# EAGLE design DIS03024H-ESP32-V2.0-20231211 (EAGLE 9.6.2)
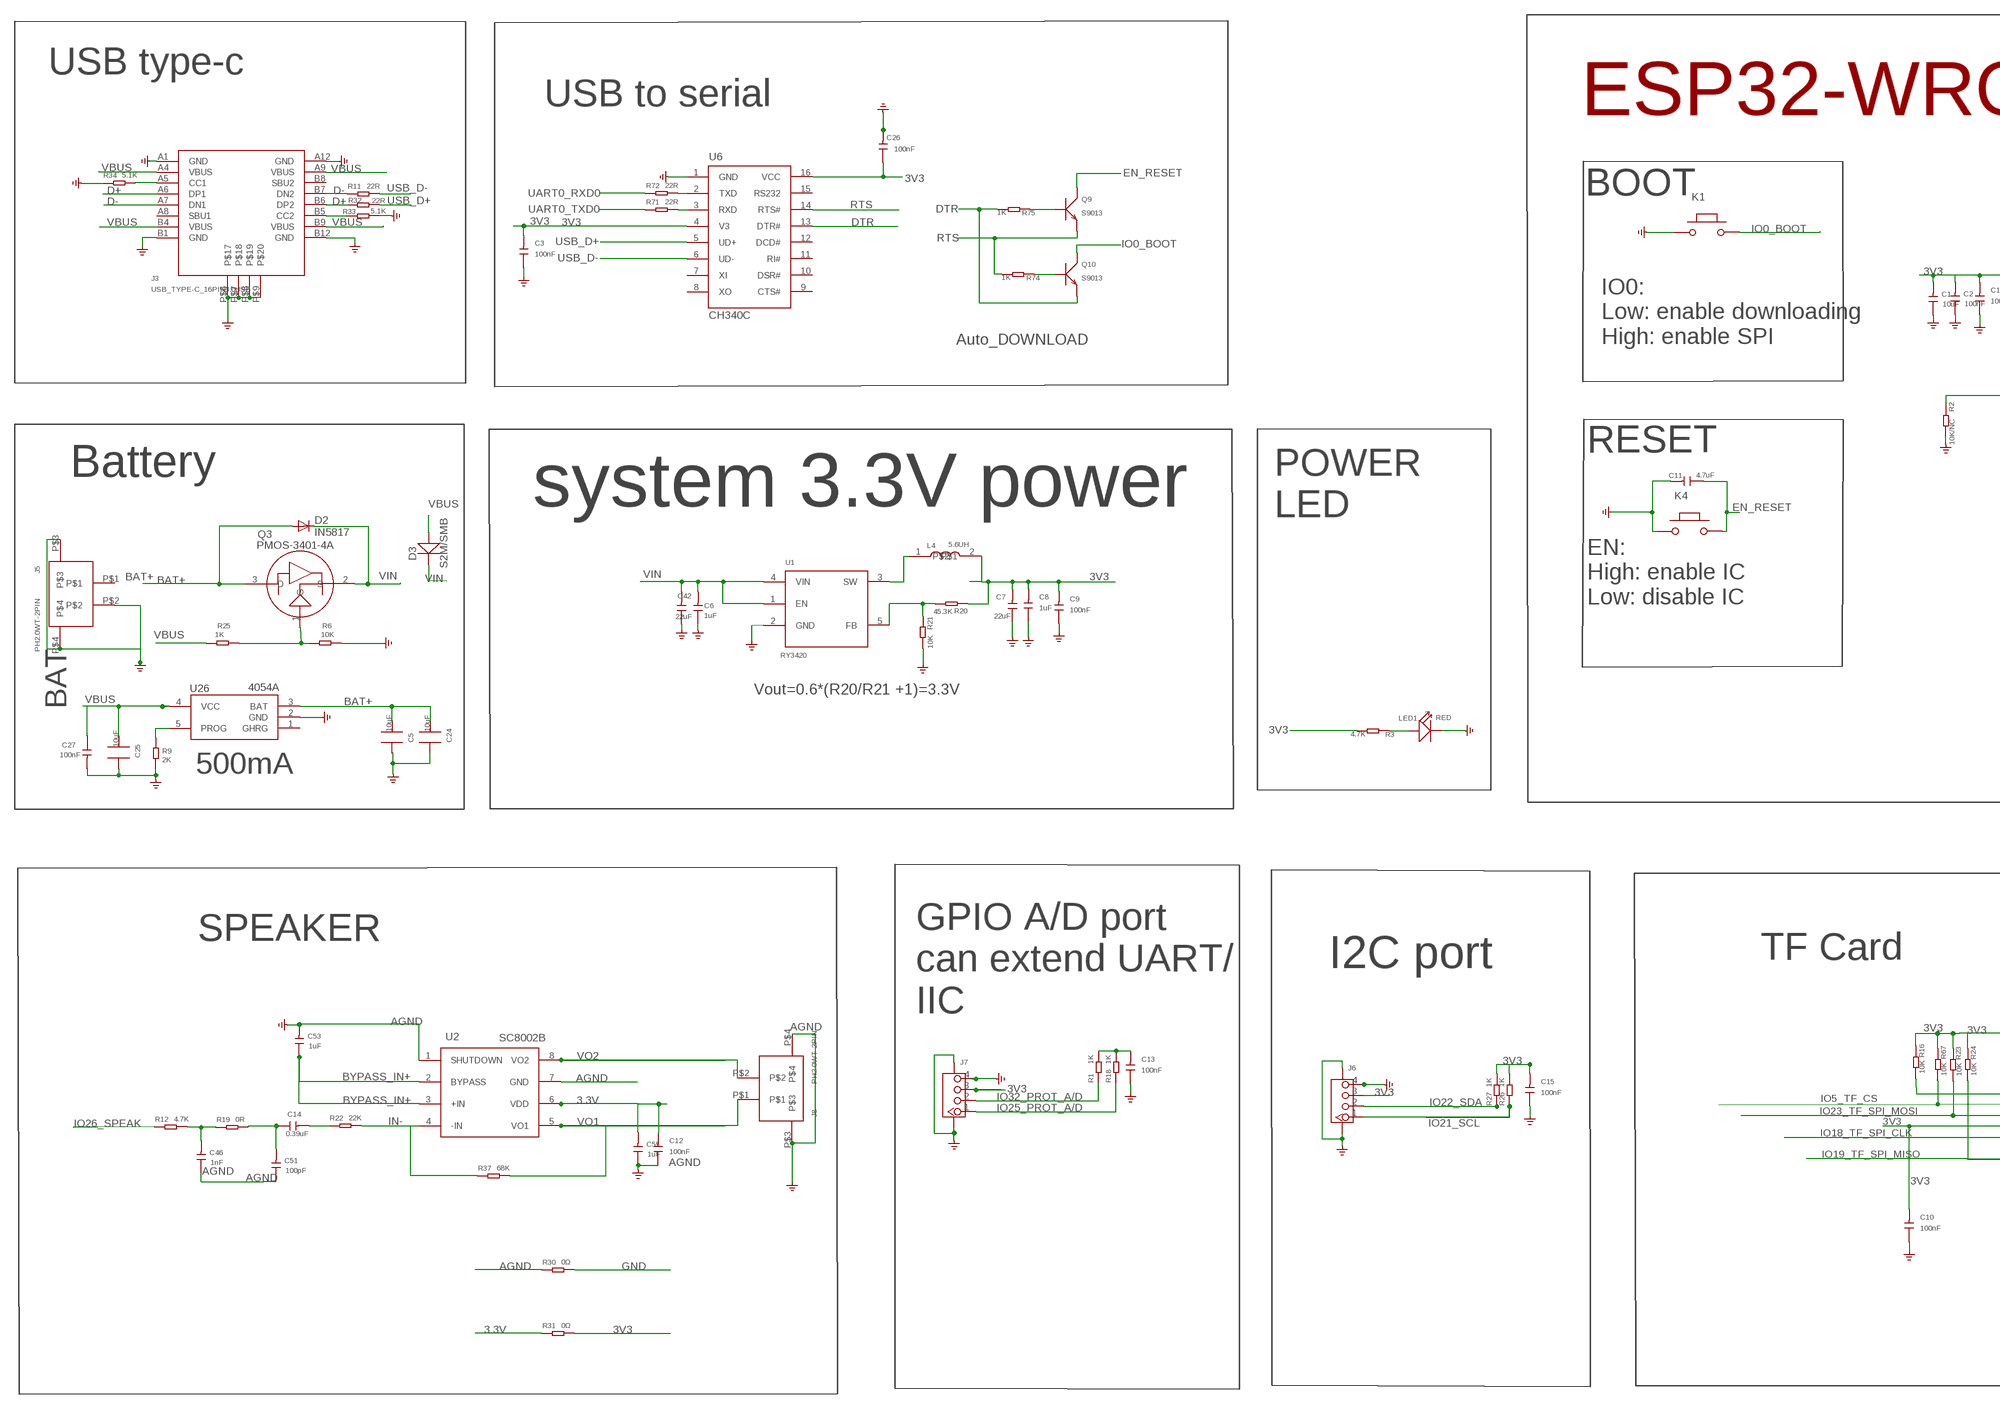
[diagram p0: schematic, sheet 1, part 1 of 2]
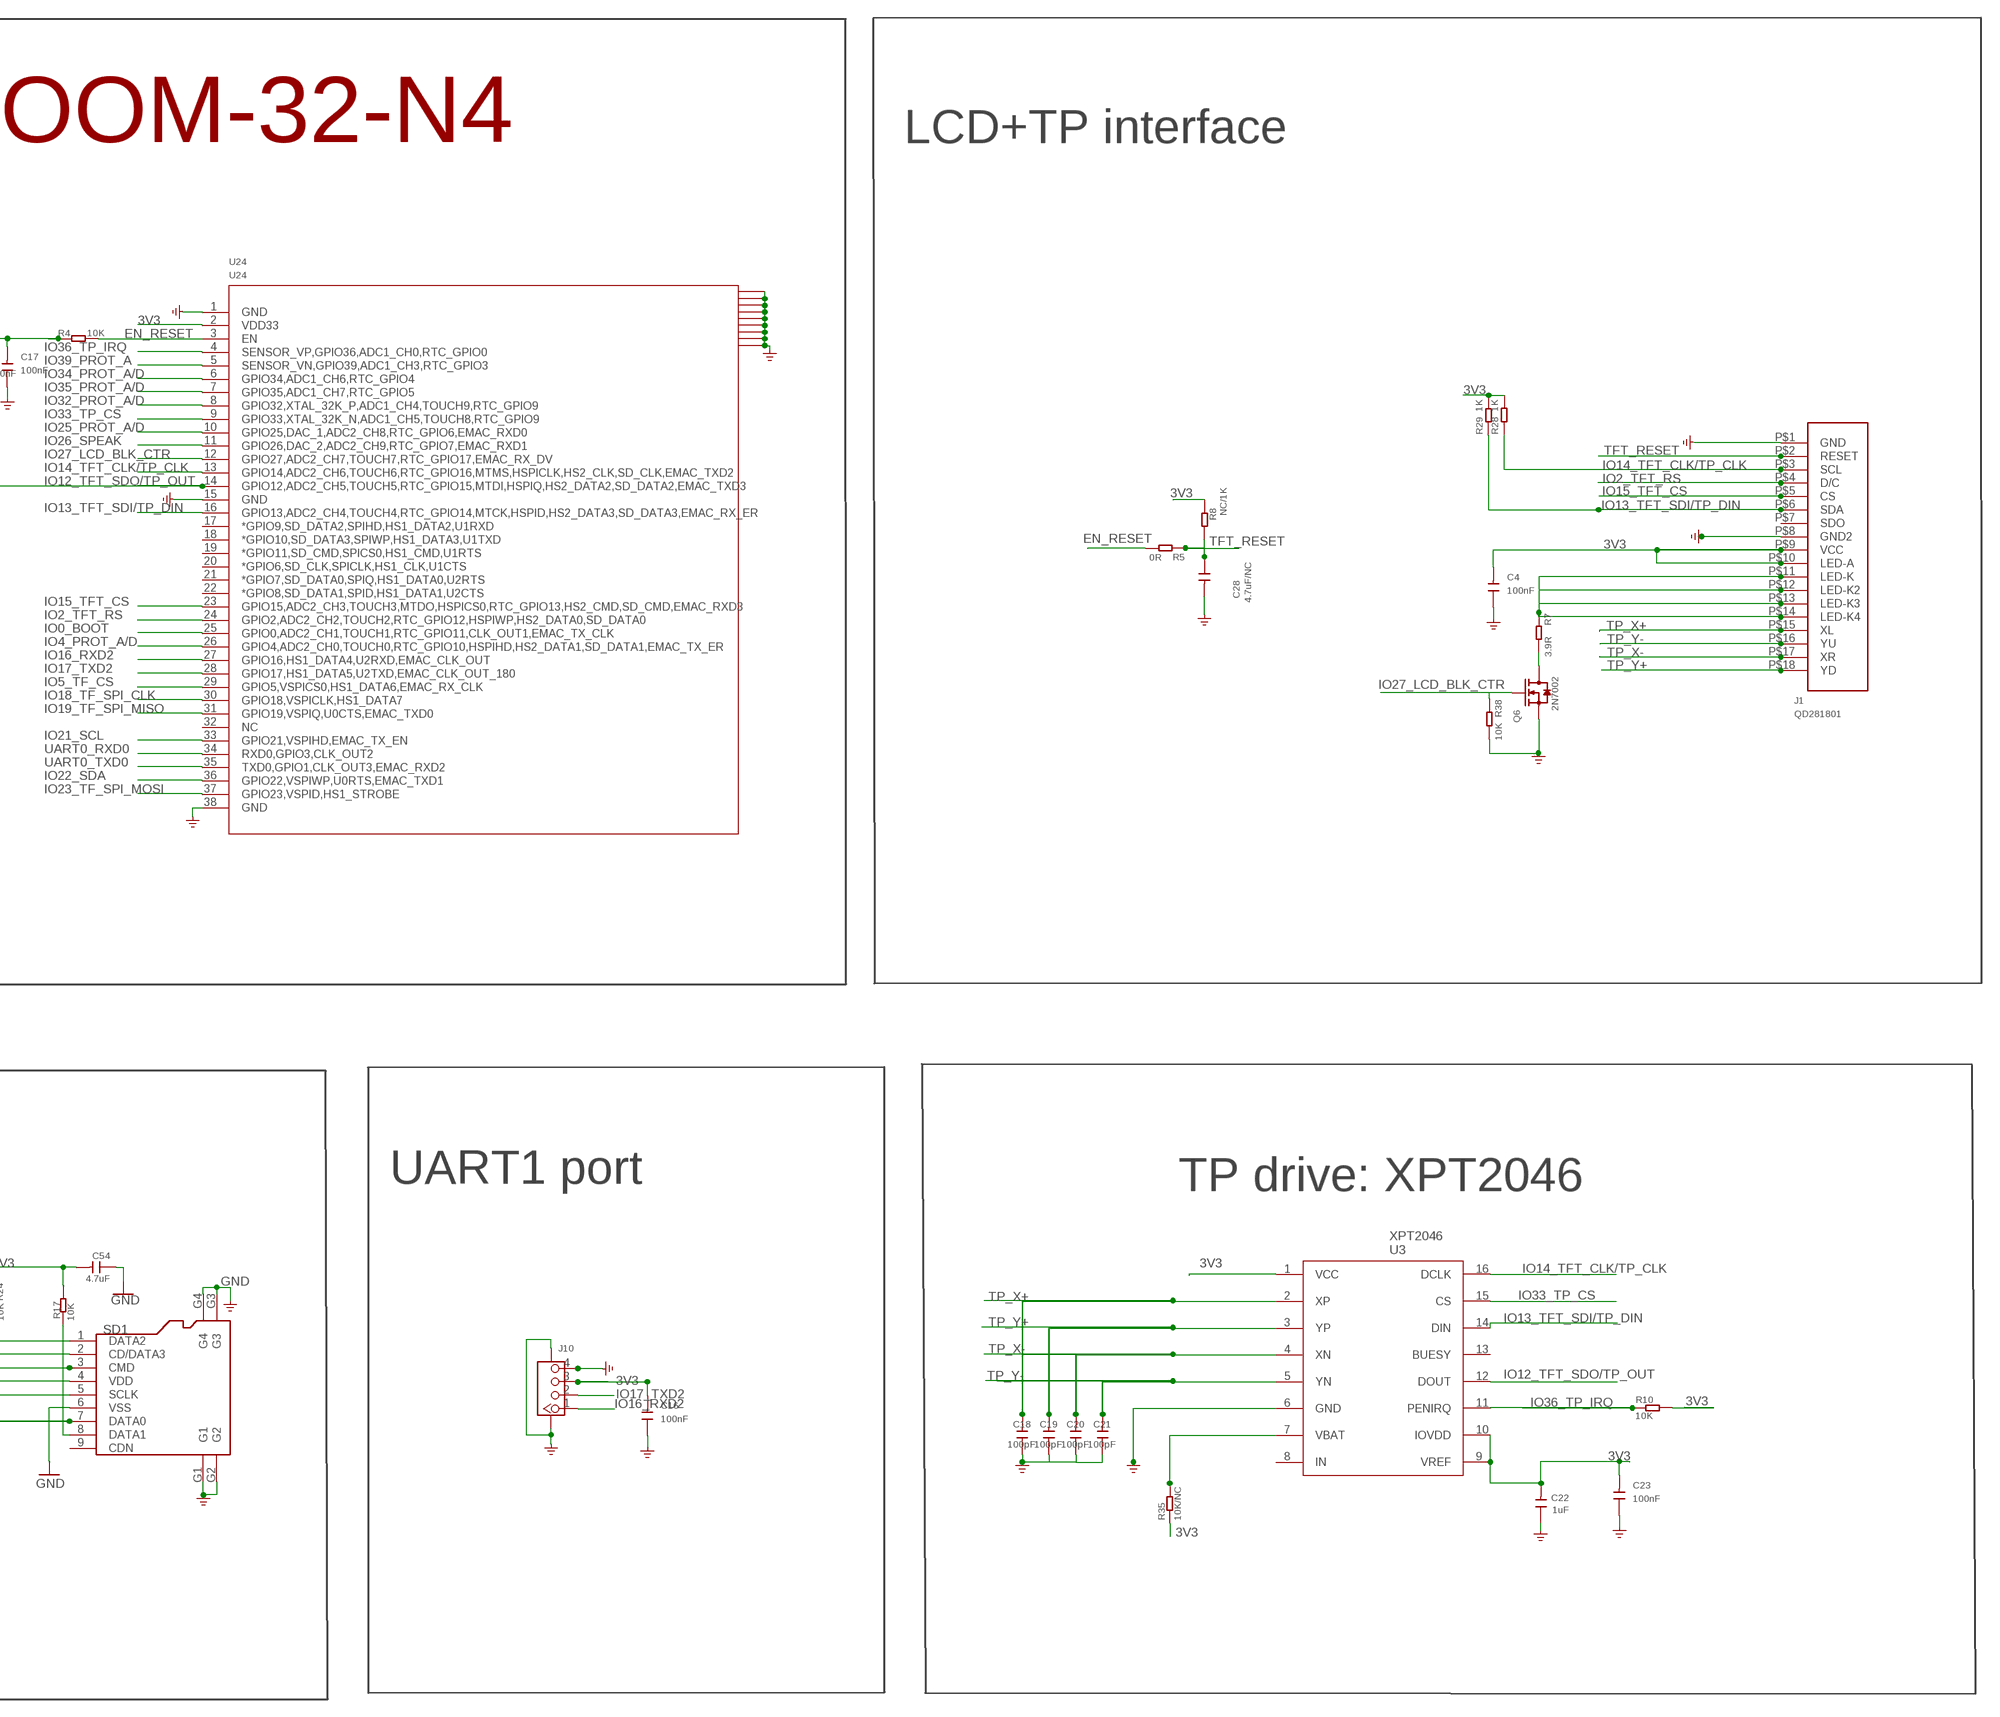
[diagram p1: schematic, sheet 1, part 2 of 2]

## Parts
C1  10uF  DISCRETE_C-0603  [DISCRETE_C0603]
C2  100nF  DISCRETE_C-0603  [DISCRETE_C0603]
C3  100nF  C0603  [0603]
C4  100nF  C0603  [0603]
C5  10uF  C0805_S  [0805_S]
C6  1uF  C0603  [0603]
C7  22uF  C0805  [0805]
C8  1uF  C0603  [0603]
C9  100nF  C0603  [0603]
C10  100nF  C0603  [0603]
C11  4.7uF  C0603  [0603]
C12  100nF  C0603  [0603]
C13  100nF  C0603  [0603]
C14  0.39uF  DISCRETE_C-0603  [DISCRETE_C0603]
C15  100nF  C0603  [0603]
C16  100nF  C0603  [0603]
C17  100nF  C0603  [0603]
C18  100pF  C0603  [0603]
C19  100pF  C0603  [0603]
C20  100pF  C0603  [0603]
C21  100pF  C0603  [0603]
C22  1uF  DISCRETE_C-0603  [DISCRETE_C0603]
C23  100nF  C0603  [0603]
C24  10uF  C0805_S  [0805_S]
C25  10uF  C0805_S  [0805_S]
C26  100nF  C0603  [0603]
C27  100nF  C-0603  [C0603]
C28  4.7uF/NC  C0603  [0603]
C42  22uF  C0805  [0805]
C46  1nF  DISCRETE_C-0603  [DISCRETE_C0603]
C51  100pF  DISCRETE_C-0603  [DISCRETE_C0603]
C53  1uF  DISCRETE_C-0603  [DISCRETE_C0603]
C54  4.7uF  DISCRETE_C-0603  [DISCRETE_C0603]
C55  1uF  DISCRETE_C-0603  [DISCRETE_C0603]
D2  IN5817  DIODE-DO-214AC  [DO-214AC]
D3  S2M/SMB  214ABDO-214AB  [214AB]
J1  QD281801  [QD241801-18PIN*0.8]
J3  USB_TYPE-C_16PIN3.0USB  [KEVIN_3.0TYPEC-SMD]
J5  PH2.0WT-2PIN  [PH2.0WT-2PIN]
J6  CONNECTOR_TWIG-4P-2.0-SMD-FEMALE-REINFORCE90D  [CONNECTOR_4P-SMD-2.0-90D]
J7  CONNECTOR_TWIG-4P-2.0-SMD-FEMALE-REINFORCE90D  [CONNECTOR_4P-SMD-2.0-90D]
J8  PH2.0WT-2PIN  [PH2.0WT-2PIN]
J10  CONNECTOR_TWIG-4P-2.0-SMD-FEMALE-REINFORCE90D  [CONNECTOR_4P-SMD-2.0-90D]
K1  BUTTON  PB157  [157SW]
K4  BUTTON  PB157  [157SW]
L4  5.6UH  L-0530  [CD54_CD54]
LED1  RED  DISCRETE_LED0603  [DISCRETE_LED-0603]
Q3  PMOS-3401-4A  P-MOS-SOT23  [SOT-23]
Q6  2N7002  MOSFET-N'SOT23'  [SOT23]
Q9  S9013  TRANSISTOR-NPN-SOT23  [SOT23@1]
Q10  S9013  TRANSISTOR-NPN-SOT23  [SOT23@1]
R1  1K  DISCRETE_R-0603  [DISCRETE_R0603]
R2  10K/NC  DISCRETE_R-0603  [DISCRETE_R0603]
R3  4.7K  DISCRETE_R-0603  [DISCRETE_R0603]
R4  10K  R0603  [R0603]
R5  0R  DISCRETE_R-0603  [DISCRETE_R0603]
R6  10K  DISCRETE_R-0603  [DISCRETE_R0603]
R7  3.9R  DISCRETE_R-0603  [DISCRETE_R0603]
R8  NC/1K  DISCRETE_R-0603  [DISCRETE_R0603]
R9  2K  DISCRETE_R-0603  [DISCRETE_R0603]
R10  10K  DISCRETE_R-0603  [DISCRETE_R0603]
R11  22R  DISCRETE_R-0603  [DISCRETE_R0603]
R12  4.7K  DISCRETE_R-0603  [DISCRETE_R0603]
R16  10K  DISCRETE_R-0603  [DISCRETE_R0603]
R17  10K  DISCRETE_R-0603  [DISCRETE_R0603]
R18  1K  DISCRETE_R-0603  [DISCRETE_R0603]
R19  0R  DISCRETE_R-0603  [DISCRETE_R0603]
R20  45.3K  DISCRETE_R-0603  [DISCRETE_R0603]
R21  10K  DISCRETE_R-0603  [DISCRETE_R0603]
R22  22K  DISCRETE_R-0603  [DISCRETE_R0603]
R23  10K  DISCRETE_R-0603  [DISCRETE_R0603]
R24  10K  DISCRETE_R-0603  [DISCRETE_R0603]
R25  1K  DISCRETE_R-0603  [DISCRETE_R0603]
R26  1K  DISCRETE_R-0603  [DISCRETE_R0603]
R27  1K  DISCRETE_R-0603  [DISCRETE_R0603]
R28  1K  DISCRETE_R-0603  [DISCRETE_R0603]
R29  1K  DISCRETE_R-0603  [DISCRETE_R0603]
R30  0Ω  DISCRETE_R-0603  [DISCRETE_R0603]
R31  0Ω  DISCRETE_R-0603  [DISCRETE_R0603]
R32  22R  DISCRETE_R-0603  [DISCRETE_R0603]
R33  5.1K  DISCRETE_R-0603  [DISCRETE_R0603]
R34  5.1K  DISCRETE_R-0603  [DISCRETE_R0603]
R35  10K/NC  DISCRETE_R-0603  [DISCRETE_R0603]
R37  68K  DISCRETE_R-0603  [DISCRETE_R0603]
R38  10K  DISCRETE_R-0603  [DISCRETE_R0603]
R67  10K  DISCRETE_R-0603  [DISCRETE_R0603]
R71  22R  DISCRETE_R-0603  [DISCRETE_R0603]
R72  22R  DISCRETE_R-0603  [DISCRETE_R0603]
R74  1K  DISCRETE_R-0603  [DISCRETE_R0603]
R75  1K  DISCRETE_R-0603  [DISCRETE_R0603]
SD1  HOLDER-MICROSD-9P  [9P-SMD-W/-RING]
U1  RY3420  A_XBJ_HM3420B  [A_XBJ_SOT23-5]
U2  SC8002B  SC8002BSC8002B-SOP8  [AT24C02_SOP8]
U3  XPT2046  [XP2046-SSOP16]
U6  CH340C  CH340G  [SOP-16]
U24  U24  ESP32-WROOM-32-N4  [ESP32-WROOM-32-N4]
U26  4054A  [SOP23-5]

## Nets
3.3V: C12.2 C55.2 R31.1 U2.6(VDD)
3V3: C1.2 C2.2 C3.2 C4.2 C7.2 C8.2 C9.2 C10.2 C13.2 C15.2 C16.2 C17.2 C22.2 C23.2 C26.1 C54.2 J1.P$9(VCC) J1.P$10(LED-A) J6.3 J7.3 J10.3 L4.2 R1.2 R3.2 R4.1 R8.2 R10.2 R16.1 R17.1 R18.2 R20.1 R23.1 R24.1 R26.2 R27.2 R28.2 R29.2 R31.2 R35.1 R67.1 SD1.4(VDD) U3.1(VCC) U3.9(VREF) U3.10(IOVDD) U6.4(V3) U6.16(VCC) U24.2(VDD33)
AGND: C12.1 C46.1 C51.1 C53.2 C55.1 J8.P$3 J8.P$4 R30.1 U2.1(SHUTDOWN) U2.7(GND) ; supply symbol labelled GND
BAT+: C5.2 C24.2 D2.A J5.P$1 Q3.3(D) U26.3(BAT)
BYPASS_IN+: C53.1 U2.2(BYPASS) U2.3(+IN)
D+: J3.A6(DP1) J3.B6(DP2) R32.1
D-: J3.A7(DN1) J3.B7(DN2) R11.1
DTR: Q10.2(E) R75.2 U6.13(DTR#)
EN_RESET: C11.1 K4.2 Q9.3(C) R4.2 R5.2 U24.3(EN)
GND: C1.1 C2.1 C3.1 C4.1 C5.1 C6.1 C7.1 C8.1 C9.1 C10.1 C11.2 C13.1 C15.1 C16.1 C17.1 C18.1 C19.1 C20.1 C21.1 C22.1 C23.1 C24.1 C25.1 C26.2 C27.2 C28.2 C42.1 C54.1 J1.P$1(GND) J1.P$8(GND2) J3.A1(GND) J3.A12(GND) J3.B1(GND) J3.B12(GND) J3.P$6 J3.P$7 J3.P$8 J3.P$9 J5.P$2 J5.P$3 J5.P$4 J6.4 J6.SS1 J6.SS2 J7.4 J7.SS1 J7.SS2 J10.4 J10.SS1 J10.SS2 K1.1 K4.1 LED1.- Q6.2(S) R2.2 R6.1 R9.2 R21.2 R30.2 R33.2 R34.1 R38.2 SD1.6(VSS) SD1.G1 SD1.G2 SD1.G3 SD1.G4 U1.2(GND) U3.6(GND) U6.1(GND) U24.1(GND) U24.15(GND) U24.38(GND) U24.41(GND) U24.42(GND) U24.43(GND) U24.44(GND) U24.45(GND) U24.46(GND) U24.47(GND) U24.48(GND) U24.49(GND) U26.2(GND)
IN-: R22.2 R37.1 U2.4(-IN)
IO0_BOOT: K1.2 Q10.3(C) U24.25(GPIO0,ADC2_CH1,TOUCH1,RTC_GPIO11,CLK_OUT1,EMAC_TX_CLK)
IO2_TFT_RS: J1.P$4(D/C) U24.24(GPIO2,ADC2_CH2,TOUCH2,RTC_GPIO12,HSPIWP,HS2_DATA0,SD_DATA0)
IO4_PROT_A/D: U24.26(GPIO4,ADC2_CH0,TOUCH0,RTC_GPIO10,HSPIHD,HS2_DATA1,SD_DATA1,EMAC_TX_ER)
IO5_TF_CS: R67.2 SD1.2(CD/DATA3) U24.29(GPIO5,VSPICS0,HS1_DATA6,EMAC_RX_CLK)
IO12_TFT_SDO/TP_OUT: R2.1 U3.12(DOUT) U24.14(GPIO12,ADC2_CH5,TOUCH5,RTC_GPIO15,MTDI,HSPIQ,HS2_DATA2,SD_DATA2,EMAC_TXD3)
IO13_TFT_SDI/TP_DIN: J1.P$6(SDA) R29.1 U3.14(DIN) U24.16(GPIO13,ADC2_CH4,TOUCH4,RTC_GPIO14,MTCK,HSPID,HS2_DATA3,SD_DATA3,EMAC_RX_ER)
IO14_TFT_CLK/TP_CLK: J1.P$3(SCL) R28.1 U3.16(DCLK) U24.13(GPIO14,ADC2_CH6,TOUCH6,RTC_GPIO16,MTMS,HSPICLK,HS2_CLK,SD_CLK,EMAC_TXD2)
IO15_TFT_CS: J1.P$5(CS) U24.23(GPIO15,ADC2_CH3,TOUCH3,MTDO,HSPICS0,RTC_GPIO13,HS2_CMD,SD_CMD,EMAC_RXD3)
IO16_RXD2: J10.1 U24.27(GPIO16,HS1_DATA4,U2RXD,EMAC_CLK_OUT)
IO17_TXD2: J10.2 U24.28(GPIO17,HS1_DATA5,U2TXD,EMAC_CLK_OUT_180)
IO18_TF_SPI_CLK: SD1.5(SCLK) U24.30(GPIO18,VSPICLK,HS1_DATA7)
IO19_TF_SPI_MISO: R24.2 SD1.7(DATA0) U24.31(GPIO19,VSPIQ,U0CTS,EMAC_TXD0)
IO21_SCL: J6.1 R26.1 U24.33(GPIO21,VSPIHD,EMAC_TX_EN)
IO22_SDA: J6.2 R27.1 U24.36(GPIO22,VSPIWP,U0RTS,EMAC_TXD1)
IO23_TF_SPI_MOSI: R23.2 SD1.3(CMD) U24.37(GPIO23,VSPID,HS1_STROBE)
IO25_PROT_A/D: J7.1 R18.1 U24.10(GPIO25,DAC_1,ADC2_CH8,RTC_GPIO6,EMAC_RXD0)
IO26_SPEAK: R12.1 U24.11(GPIO26,DAC_2,ADC2_CH9,RTC_GPIO7,EMAC_RXD1)
IO27_LCD_BLK_CTR: Q6.1(G) R38.1 U24.12(GPIO27,ADC2_CH7,TOUCH7,RTC_GPIO17,EMAC_RX_DV)
IO32_PROT_A/D: J7.2 R1.1 U24.8(GPIO32,XTAL_32K_P,ADC1_CH4,TOUCH9,RTC_GPIO9)
IO33_TP_CS: U3.15(CS) U24.9(GPIO33,XTAL_32K_N,ADC1_CH5,TOUCH8,RTC_GPIO9)
IO34_PROT_A/D: U24.6(GPIO34,ADC1_CH6,RTC_GPIO4)
IO35_PROT_A/D: U24.7(GPIO35,ADC1_CH7,RTC_GPIO5)
IO36_TP_IRQ: R10.1 U3.11(PENIRQ) U24.4(SENSOR_VP,GPIO36,ADC1_CH0,RTC_GPIO0)
IO39_PROT_A: U24.5(SENSOR_VN,GPIO39,ADC1_CH3,RTC_GPIO3)
N$1: LED1.+ R3.1
N$2: Q6.3(D) R7.2
N$3: C46.2 R12.2 R19.1
N$4: R35.2 U3.7(VBAT)
N$6: R9.1 U26.5(PROG)
N$12: J1.P$11(LED-K) J1.P$12(LED-K2) J1.P$13(LED-K3) J1.P$14(LED-K4) R7.1
N$13: L4.1 U1.3(SW)
N$14: J3.B5(CC2) R33.1
N$16: J3.A5(CC1) R34.2
N$17: Q3.1(G) R6.2 R25.1
N$20: R20.2 R21.1 U1.5(FB)
N$26: C14.1 C51.2 R19.2
N$29: C14.2 R22.1
N$32: Q9.1(B) R75.1
N$38: Q10.1(B) R74.1
N$40: R72.2 U6.2(TXD)
N$42: R71.2 U6.3(RXD)
N$47: R16.2 SD1.1(DATA2)
N$48: R17.2 SD1.8(DATA1)
RTS: Q9.2(E) R74.2 U6.14(RTS#)
TFT_RESET: C28.1 J1.P$2(RESET) R5.1 R8.1
TP_X+: C18.2 J1.P$15(XL) U3.2(XP)
TP_X-: C20.2 J1.P$17(XR) U3.4(XN)
TP_Y+: C19.2 J1.P$18(YD) U3.3(YP)
TP_Y-: C21.2 J1.P$16(YU) U3.5(YN)
UART0_RXD0: R72.1 U24.34(RXD0,GPIO3,CLK_OUT2)
UART0_TXD0: R71.1 U24.35(TXD0,GPIO1,CLK_OUT3,EMAC_RXD2)
USB_D+: R32.2 U6.5(UD+)
USB_D-: R11.2 U6.6(UD-)
VBUS: C25.2 C27.1 D3.1(+) J3.A4(VBUS) J3.A9(VBUS) J3.B4(VBUS) J3.B9(VBUS) R25.2 U26.4(VCC)
VIN: C6.2 C42.2 D2.C D3.2(-) Q3.2(S) U1.1(EN) U1.4(VIN)
VO1: J8.P$1 R37.2 U2.5(VO1)
VO2: J8.P$2 U2.8(VO2)
Unconnected: J1.P$7(SDO) J3.A8(SBU1) J3.B8(SBU2) SD1.9(CDN) U3.8(IN) U3.13(BUESY) U6.7(XI) U6.8(XO) U6.9(CTS#) U6.10(DSR#) U6.11(RI#) U6.12(DCD#) U6.15(RS232) U24.17(*GPIO9,SD_DATA2,SPIHD,HS1_DATA2,U1RXD) U24.18(*GPIO10,SD_DATA3,SPIWP,HS1_DATA3,U1TXD) U24.19(*GPIO11,SD_CMD,SPICS0,HS1_CMD,U1RTS) U24.20(*GPIO6,SD_CLK,SPICLK,HS1_CLK,U1CTS) U24.21(*GPIO7,SD_DATA0,SPIQ,HS1_DATA0,U2RTS) U24.22(*GPIO8,SD_DATA1,SPID,HS1_DATA1,U2CTS) U24.32(NC) U26.1(GHRG)

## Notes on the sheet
- USB type-c
- USB to serial | ESP32-WROOM-32-N4 | LCD+TP interface
- BOOT
- IO0:
  Low: enable downloading
  High: enable SPI
- Auto_DOWNLOAD
- RESET
- Battery
- system 3.3V power
- POWER
  LED
- EN:
  High: enable IC
  Low: disable IC
- Vout=0.6*(R20/R21 +1)=3.3V
- BAT
- 500mA
- SPEAKER
- I2C port | TF Card | UART1 port
- TP drive: XPT2046
- GPIO A/D port
  can extend UART/
  IIC

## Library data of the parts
C1 C2 C14 C22 C46 C51 C53 C55 = A_xbj:DISCRETE_C*: Ceramic Capacitors
C3 C4 C6 C8-C13 C15-C21 C23 C26 C28 = A_xbj:C0603
C5 C24 C25 = CPT_SMD:C0805
C7 C42 = A_xbj:C0805
C27 = discrete:C*: Ceramic Capacitors
C54 = A9G:DISCRETE_C*: Ceramic Capacitors
D2 = diode:DIODE-: DIODE
D3 = DO-214AB:214AB: 214AB
J1 = cooper:QD281801
J3 = WZ3532R024-ESP32-V0.1-20221226:USB_TYPE-C_16PIN
J5 J8 = cooper:PH2.0WT-2PIN
J6 J7 J10 = A_xbj:CONNECTOR_TWIG-4P-2.0-SMD-FEMALE-REINFORCE
K1 K4 = MySMD:PB157
L4 = WZ2432R028-ESP32-V1.2-20231108:L-0530
LED1 = A_xbj:DISCRETE_LED*
Q3 = DFN8:P-MOS-SOT23
Q6 = discrete:MOSFET-N: IRLL014: http://www.vishay.com/docs/91319/sihll014.pdf
Q9 Q10 = discrete:TRANSISTOR-NPN*: NPN audion
R1-R3 R5 R7 R8 R11 R12 R16-R24 R26-R34 R37 R38 R67 R71 R72 R74 R75 = Crowtail-_LED-V2.0-20190615-01:DISCRETE_R*
R4 = A_xbj:R0603
R6 R9 R10 R25 R35 = A9G:DISCRETE_R*
SD1 = Connector:HOLDER-MICROSD-9P
U1 = CrowBot_-V1.0-20220525:A_XBJ_HM3420B
U2 = cooper:SC8002B
U3 = cooper:XPT2046
U6 = A_xbj:CH340G
U24 = cooper:ESP32-WROOM-32-N4
U26 = DFN8:4054A

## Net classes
0 default: width 0.152 mm, drill 0.305 mm, clearance 0.203 mm

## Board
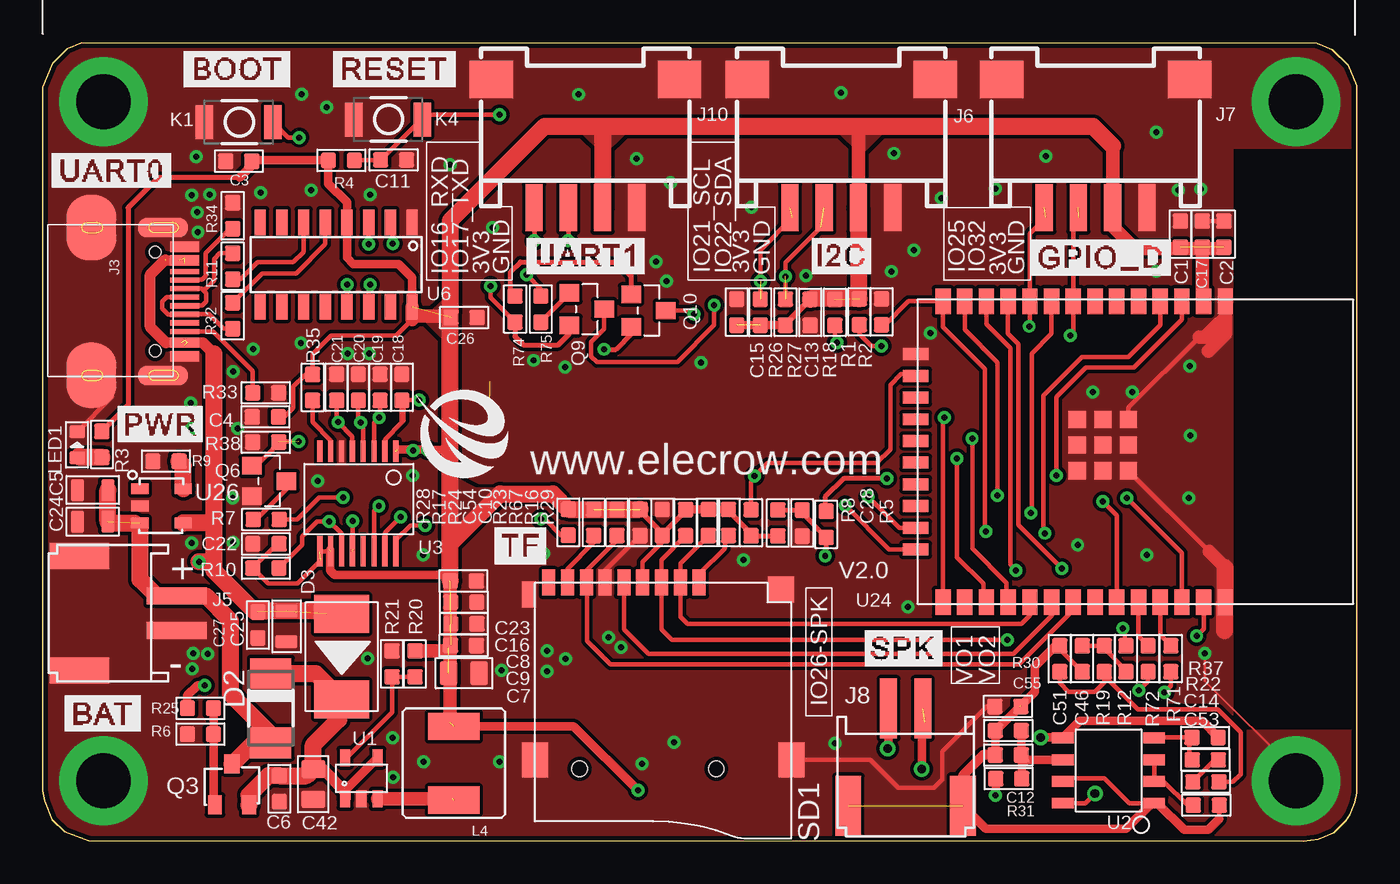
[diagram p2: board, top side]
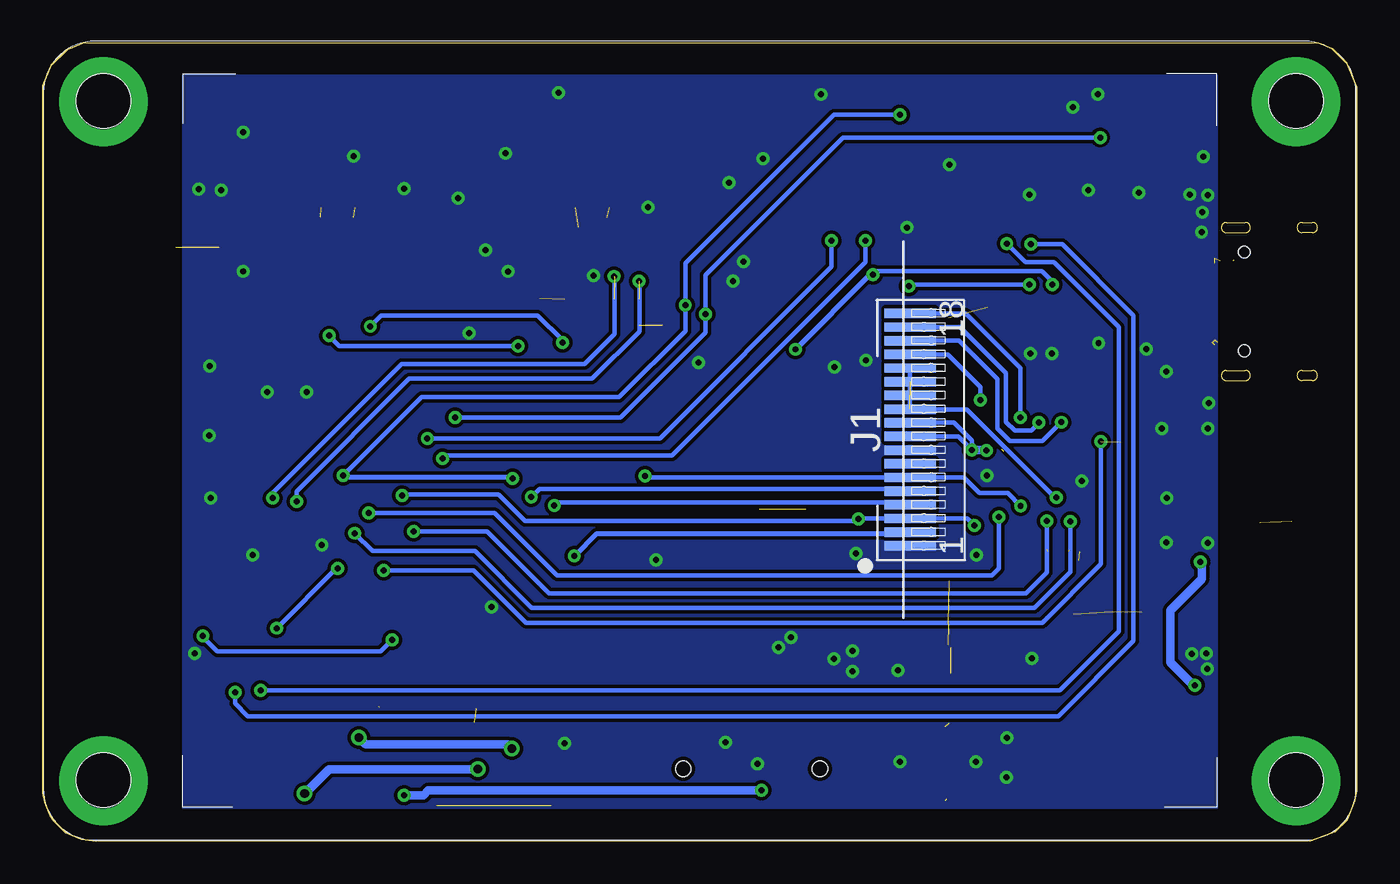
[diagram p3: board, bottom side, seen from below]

Size 76.85 x 46.71 mm. Coordinates in mm from the lower left corner, seen from the top.
Outline: 2.27,46.71 74.52,46.69 75.43,46.31 76.35,45.38 76.85,44.18 76.85,2.84 76.74,2.26 76.44,1.54 76.2,1.18 75.52,0.5 74.61,0.13 73.72,0 2.68,0.02 1.28,0.55 0.57,1.27 0.11,2.36 0,2.94 0,44.11 0.58,45.52 1.42,46.36 2.27,46.71
Copper layers (1*16): Top 0.035mm / dielectric 1.5mm / Bottom 0.035mm
Design rules "default *": minimum track width 6mil, minimum drill 0.35mm, track to track 6mil, track to pad 5mil, pad to pad 5mil, via to via 6mil, smd to smd 6mil, copper to edge 10mil, drill to drill 10mil, minimum pad ring 10mil, minimum via ring 8mil, stop-mask expansion 4mil, vias tented up to drill 100mil, thermal gap 0mil
tRestrict: area 22.3,131.3 to 32.1,150.4
bRestrict: area 22.3,131.3 to 32.1,150.4

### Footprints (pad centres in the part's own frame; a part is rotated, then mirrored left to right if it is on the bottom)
DISCRETE_C0603 = smd 0.889 x 0.889: 1 -0.762,0; 2 0.762,0
0603 = smd 0.889 x 0.889: 1 -0.762,0; 2 0.762,0
0805_S = smd 0.762 x 1.27: 1 -0.889,0; 2 0.889,0
0805 = smd 1.016 x 1.397: 1 -0.889,0; 2 0.889,0
C0603 = smd 0.889 x 0.889: 1 -0.762,0; 2 0.762,0
DO-214AC = smd 1.8 x 2.4: A 2.025,0; C -2.025,0
214AB = smd 2.2 x 3.2: 1 -2.5,0; 2 2.5,0
QD241801-18PIN*0.8 = smd 0.55 x 3: P$1 -6.789,-1.538; P$2 -5.989,-1.538; P$3 -5.189,-1.538; P$4 -4.389,-1.538; P$5 -3.589,-1.538; P$6 -2.789,-1.538; P$7 -1.989,-1.538; P$8 -1.189,-1.538; P$9 -0.389,-1.538; P$10 0.411,-1.538; P$11 1.211,-1.538; P$12 2.011,-1.538; P$13 2.811,-1.538; P$14 3.611,-1.538; P$15 4.411,-1.538; P$16 5.211,-1.538; P$17 6.011,-1.538; P$18 6.811,-1.538
KEVIN_3.0TYPEC-SMD = smd 0.3 x 1.7: A1 -3.35,0.5; A4 -2.55,0.5; A5 -1.25,0.5; A6 -0.25,0.5; A7 0.25,0.5; A8 1.25,0.5; A9 2.55,0.5; A12 3.35,0.5; B1 3.05,0.5; B4 2.25,0.5; B5 1.75,0.5; B6 0.75,0.5; B7 -0.75,0.5; B8 -1.75,0.5; B9 -2.25,0.5; B12 -3.05,0.5 | smd 1.143 x 2.921: P$6 -4.318,-0.762; P$7 4.318,-0.762 | smd 3.81 x 2.921: P$8 -4.318,-4.953; P$9 4.318,-4.953 | hole 0.68: -2.89,-1.22; 2.89,-1.22
PH2.0WT-2PIN = smd 1 x 3.5: P$1 -1,0; P$2 1,0 | smd 1.5 x 3.5: P$3 -3.35,-5.7; P$4 3.35,-5.7
CONNECTOR_4P-SMD-2.0-90D = smd 1.01 x 2.74: 1 -3,-0.1; 2 -1,-0.1; 3 1,-0.1; 4 3,-0.1 | smd 2.54 x 2.184: SS1 -5.5,7.4; SS2 5.5,7.4
157SW = smd 1.016 x 1.981: 1 0,0; 2 4,0
CD54_CD54 = smd 3 x 1.6: 1 0,2.159; 2 0,-2.159
DISCRETE_LED-0603 = smd 0.762 x 0.889: + -0.762,0; - 0.762,0
SOT-23 = smd 1.1 x 0.8: 1 1.2,-1; 2 1.2,1 | smd 1.1 x 0.9: 3 -1.2,0
SOT23 = smd 1.016 x 1.143: 1 -0.889,-1.016; 2 0.889,-1.016; 3 0,1.016
SOT23@1 = smd 1.016 x 1.143: 1 -0.95,-1.016; 2 0.95,-1.016; 3 0,1.016
DISCRETE_R0603 = smd 0.889 x 0.889: 1 -0.762,0; 2 0.762,0
R0603 = smd 0.889 x 0.889: 1 -0.762,0; 2 0.762,0
9P-SMD-W/-RING = smd 1.524 x 0.762: 1 0,4.4; 2 0,3.3; 3 0,2.2; 4 0,1.1; 5 0,0; 6 0,-1.1; 7 0,-2.2; 8 0,-3.3; 9 0,-4.4 | smd 1.524 x 0.8: G1 0.7,-5.546 | smd 2.032 x 1.524: G2 10.373,-5.2; G3 10.373,9.8 | smd 1.524 x 1.524: G4 0.392,9.181 | hole 0.889: 10.9,-2.6; 10.9,5.4
A_XBJ_SOT23-5 = smd 0.6 x 1: 1 -0.95,-1.2; 2 0,-1.2; 3 0.95,-1.2; 4 0.95,1.2; 5 -0.95,1.2
AT24C02_SOP8 = smd 0.635 x 1.27: 1 -1.905,-2.667; 2 -0.635,-2.667; 3 0.635,-2.667; 4 1.905,-2.667; 5 1.905,2.667; 6 0.635,2.667; 7 -0.635,2.667; 8 -1.905,2.667
XP2046-SSOP16 = smd 0.305 x 1.27: 1 -2.54,-2.54; 2 -1.905,-2.54; 3 -1.27,-2.54; 4 -0.635,-2.54; 5 0,-2.54; 6 0.635,-2.54; 7 1.27,-2.54; 8 1.905,-2.54 | smd 0.305 x 1.778: 9 1.905,3.302; 10 1.27,3.302; 11 0.635,3.302; 12 0,3.302; 13 -0.635,3.302; 14 -1.27,3.302; 15 -1.905,3.302; 16 -2.54,3.302
SOP-16 = smd 0.66 x 1.5: 1 -4.445,-2.475; 2 -3.175,-2.475; 3 -1.905,-2.475; 4 -0.635,-2.475; 5 0.635,-2.475; 6 1.905,-2.475; 7 3.175,-2.475; 8 4.445,-2.475; 9 4.445,2.475; 10 3.175,2.475; 11 1.905,2.475; 12 0.635,2.475; 13 -0.635,2.475; 14 -1.905,2.475; 15 -3.175,2.475; 16 -4.445,2.475
ESP32-WROOM-32-N4 = smd 1.5 x 0.9: 1 -8.898,6.761; 2 -8.898,5.491; 3 -8.898,4.221; 4 -8.898,2.951; 5 -8.898,1.681; 6 -8.898,0.411; 7 -8.898,-0.859; 8 -8.898,-2.129; 9 -8.898,-3.399; 10 -8.898,-4.669; 11 -8.898,-5.939; 12 -8.898,-7.209; 13 -8.898,-8.479; 14 -8.898,-9.749; 25 8.702,-9.749; 26 8.702,-8.479; 27 8.702,-7.209; 28 8.702,-5.939; 29 8.702,-4.669; 30 8.702,-3.399; 31 8.702,-2.129; 32 8.702,-0.859; 33 8.702,0.411; 34 8.702,1.681; 35 8.702,2.951; 36 8.702,4.221; 37 8.702,5.491; 38 8.702,6.761 | smd 0.7 x 1.5: 15 -5.808,-11.349; 16 -4.538,-11.349; 17 -3.268,-11.349; 18 -1.998,-11.349; 19 -0.728,-11.349; 20 0.542,-11.349; 21 1.812,-11.349; 22 3.082,-11.349; 23 4.352,-11.349; 24 5.622,-11.349 | smd 1 x 1: 41 -0.484,-0.402; 42 1.016,-0.402; 43 -1.984,-0.402; 44 -1.984,-1.902; 45 -0.484,-1.902; 46 1.016,-1.902; 47 1.016,1.098; 48 -0.484,1.098; 49 -1.984,1.098
SOP23-5 = smd 1 x 0.635: 1 -1.27,1; 2 -1.27,0; 3 -1.27,-1; 4 1.27,-1; 5 1.27,1

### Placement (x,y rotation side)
C1  66.54,35.51 270 top
C2  69.08,35.51 270 top
C3  11.47,39.78 0 top
C4  13.02,24.82 0 top
C5  2.92,20.54 0 top
C6  13.84,3.07 90 top
C7  24.63,9.83 180 top
C8  24.63,12.72 180 top
C9  24.61,11.45 180 top
C10  36.23,18.64 270 top
C11  20.52,39.85 0 top
C12  56.47,5.04 0 top
C13  44.88,30.94 90 top
C14  68.03,3.47 180 top
C15  40.59,30.95 270 top
C16  24.63,13.98 180 top
C17  67.81,35.51 270 top
C18  21,26.55 270 top
C19  19.73,26.55 270 top
C20  18.46,26.55 270 top
C21  17.19,26.55 270 top
C22  13.05,17.39 0 top
C23  24.6,15.23 180 top
C24  2.92,18.7 0 top
C25  14.26,12.56 90 top
C26  24.65,30.63 0 top
C27  12.58,12.65 270 top
C28  44.42,18.61 270 top
C42  15.82,3.33 90 top
C46  60.79,10.67 90 top
C51  59.48,10.67 270 top
C53  68.05,2.11 0 top
C54  34.94,18.64 90 top
C55  56.47,6.47 0 top
D2  13.34,7.78 270 top
D3  17.48,10.8 270 top
J1  27.66,24.07 90 bottom
J3  7.79,31.57 270 top
J5  7.84,13.34 270 top
J6  46.7,37.16 0 top
J7  61.57,37.16 0 top
J8  50.47,7.78 0 top
J10  31.74,37.16 0 top
K1  9.46,42.06 0 top
K4  18.2,42.21 0 top
L4  24.04,4.56 180 top
LED1  2.01,23.19 90 top
Q3  11.07,3.32 270 top
Q6  13.24,21.07 270 top
Q9  31.82,31.13 270 top
Q10  35.43,31.04 270 top
R1  47.76,30.97 90 top
R2  49.06,30.97 90 top
R3  3.46,23.21 90 top
R4  17.47,39.83 0 top
R5  45.82,18.53 90 top
R6  9.22,6.26 0 top
R7  13.07,18.82 180 top
R8  42.99,18.62 270 top
R9  7.21,22.22 180 top
R10  13.05,15.97 180 top
R11  11.11,33.64 270 top
R12  63.35,10.67 270 top
R16  40.11,18.64 270 top
R17  32.22,18.64 270 top
R18  46.33,30.94 90 top
R19  62.08,10.67 270 top
R20  21.77,10.37 270 top
R21  20.42,10.37 90 top
R22  67.99,4.76 180 top
R23  37.6,18.64 270 top
R24  33.58,18.64 270 top
R25  9.22,7.78 180 top
R26  41.96,30.95 270 top
R27  43.44,30.95 270 top
R28  30.73,18.65 90 top
R29  41.42,18.63 270 top
R30  56.44,7.89 180 top
R31  56.5,3.66 180 top
R32  11.11,30.74 90 top
R33  13.05,26.23 0 top
R34  11.11,36.59 270 top
R35  15.78,26.55 270 top
R37  67.97,6.07 0 top
R38  13.05,23.34 180 top
R67  38.93,18.64 270 top
R71  65.98,10.67 270 top
R72  64.65,10.67 270 top
R74  27.62,31.13 270 top
R75  29.13,31.13 90 top
SD1  33.99,15.13 270 top
U1  18.64,3.68 0 top
U2  62.34,4.13 90 top
U3  18.11,20.27 180 top
U6  17.16,33.73 180 top
U24  62.4,22.69 270 top
U26  6.95,19.62 0 top
U$2  [2.4板框]  not placed on the board
U$30  [ELECROW-NEW]  21.8,21.25 0 top

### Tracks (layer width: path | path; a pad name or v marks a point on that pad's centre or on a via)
3.3V
  Top 0.254: R31.1 57.26,4.51 | 57.26,5.02 C12.2
  Top 0.5: U2.6 57.52,4.77 57.26,4.51 | R31.1 57.26,5.02 | C55.2 C12.2
3V3  (via drill 0.35)  (15 unrouted)
  Top 0.203: 23.74,11.35 C9.2 23.87,11.48 | C8.2 23.84,12.69
  Top 0.254: SD1.4 35.09,16.35 36.23,17.49 C10.2 | v55.71,2.69 55.73,2.69 | C22.2 13.71,17.39 R10.2 13.19,15.07 14.91,15.07 16.26,16.42 | C3.2 12.28,39.83 | U6.16 21.61,30.72 | 21.61,30.51 20.66,29.57 16.86,29.57 15.78,28.49 R35.1 15.36,27.31 14.64,26.59 14.64,25.34 14.12,24.82 C4.2 | R67.1 40.09,19.41 R16.1 | U3.9 U3.10
  Top 0.3: 36.23,18.01 34.94,19.31 | 37.6,19.33 36.23,17.97 | 41.43,18 40.11,19.32 | 11.52,38.82 6.75,38.82 4.99,37.06 4.99,25.5 R3.2 | R29.2 42.98,17.87 R8.2
  Top 0.35: 43.44,30.25 C13.2
  Top 0.5: 55.73,2.69 R31.2 | v34.81,2.97 31.05,6.72 L4.2 | C23.2 23.84,15.38 23.64,15.58 17.08,15.58 16.81,15.85 16.81,17.04 | C3.2 12.23,39.53 11.52,38.82 | 12.28,39.83 R4.1 16.7,38.48 17.8,37.39 U6.4 17.8,34.13 18.16,33.77 20.81,33.77 21.61,32.97 U6.16 | C54.2 34.94,19.31 | 37.6,19.33 R23.1 R16.1 40.11,19.32 | C10.2 36.23,17.97 36.23,18.01 | 41.43,18 R29.2 | C15.2 R27.2 43.44,30.25 | 23.57,22.88 v22.51,22.88 22.48,22.91 20.75,22.91
  Top 0.8: 23.84,6.93 C23.2 | C9.2 23.53,11.14 R20.1 | 21.61,30.51 U6.16 | J6.3 47.7,41.57 47.46,41.82 | 62.57,40.67 J7.3 62.57,35.95 63.86,34.67 69,34.67 C2.2 | C17.2 67.81,31.66 U24.2 | 23.84,30.97 23.59,30.72 21.61,30.72 | 23.57,22.88 23.84,22.62
  Top 1: C23.2 23.84,17.4 | 23.84,17.4 26.76,20.32 29.83,20.32 R28.2 C54.2 | 23.84,17.4 23.84,22.62 23.84,30.97 23.84,36.3 29.36,41.82 32.86,41.82 | 32.86,41.82 47.46,41.82 61.42,41.82 62.57,40.67 | J6.3 47.7,31.79 R1.2 44.91,31.73 C13.2 | 32.86,41.82 32.74,41.7 J10.3
  Bottom 0.254: J1.P$10 23.55,24.48 22.51,23.43 v22.51,22.88 23.3,23.68 J1.P$9 | v21.66,22.87 21.67,22.88
  Bottom 0.5: v55.71,2.69 54.59,2.69 54.31,2.97 v34.81,2.97 | 21.67,22.88 v22.51,22.88
  pour Top (no thermals): 25.36,20.67 26.86,20.67 24.26,18.07 24.16,18.07 24.16,21.27
  pour Top: 22.16,30.62 23.61,29.17 23.61,31.87 22.36,30.62
  pour Top: 32.71,40.07 34.16,41.52 31.46,41.52 32.71,40.27
  pour Top (no thermals): 47.76,40.07 49.21,41.52 46.51,41.52 47.76,40.27
AGND  (2 unrouted)
  Top 0.254: C46.1 59.48,11.23 C51.1 59.48,11.48 | 57.07,7.89 R30.1 | C53.2 68.81,1.32 | U2.1 63.55,2.23 62.09,3.69 59.85,3.69 U2.7 | J8.P$4 53.82,3.85
  Top 0.5: C51.1 59.39,11.52 59.31,11.52 58.02,10.24 58.02,8.74 57.16,7.87 | C12.1 C55.1 55.76,6.47 57.17,7.89 R30.1 | 68.81,1.32 68.16,0.67 66.76,0.67 65.2,2.23 U2.1 64.86,2.23 63.35,0.72 55.17,0.72 J8.P$4
  Top 0.58: C12.1 55.01,5.04 53.82,3.85
BAT+  (1 unrouted)
  Top 1: Q3.3 11.09,4.51 12.33,5.75 D2.A 13.58,5.75 13.93,6.1 13.48,6.1 10.97,8.61 10.97,12.91 9.55,14.34 J5.P$1 6.67,14.34 5.69,15.31 5.69,18.28 5.37,18.6 3.91,18.6 C24.2 C5.2
BYPASS_IN+
  Top 0.254: U2.3 U2.2 65.02,3.52 65.53,3.52 66.98,2.06 67.23,2.06 C53.1
D+
  Top 0.254: R32.1 10.58,29.98 9.74,30.82 J3.B6 7.33,30.82 6.99,31.15 6.99,31.57 7.25,31.82 J3.A6
D-
  Top 0.254: J3.B7 9.29,32.32 9.3,32.33 9.42,32.2 | R11.1 10.36,34.4 10.02,34.06 10.02,32.8 9.42,32.2 | J3.A7 9.31,31.32 9.56,31.57 9.56,32.07 9.42,32.2
DTR  (via drill 0.35)
  Top 0.254: U6.13 v17.8,32.55 v17.79,32.56 | v28.29,33.14 29.21,32.22 29.21,31.97 R75.2
  Top 0.3: Q10.2 34.41,29.67 33.52,28.78 v32.83,28.78
  Bottom 0.254: v17.79,32.56 17.79,32.72 18.4,33.34 28.1,33.34 v28.29,33.14
  Bottom 0.3: v32.83,28.78 28.46,33.14 v28.29,33.14
EN_RESET  (via drill 0.35)
  Top 0.254: U24.3 66.63,31.57 66.63,30.52 63.82,27.7 60.99,27.7 59.27,25.98 v59.27,21.41 | C11.1 18.26,39.85 R4.2 | C11.1 22.12,42.22 K4.2 | C11.1 22.41,42.51 v26.72,42.51 | Q9.3 32.83,29.95 32.08,29.2 32.08,28.36 32.41,28.02 37.11,28.02 39.27,30.18 v39.27,31.36
  Top 0.3: v49.37,21.22 | v49.37,21.22 46.85,21.22 45.76,20.12 45.76,19.35 R5.2
  Bottom 0.254: v59.27,21.41 54.7,25.98 43.14,25.98 39.27,29.84 v39.27,31.36 39.27,33.81 30.58,42.51 v26.72,42.51
  Bottom 0.3: v59.27,21.41 59.16,21.29 49.45,21.29 v49.37,21.22
GND  (via drill 0.35, 3.2 pad 5.2)
  Top 0.152: v67.97,10.99 67.97,9.39 73.3,4.06 v73.3,3.53
  Top 0.254: SD1.6 32.89,15.83 C54.1 | SD1.G3 48.41,4.76 50.06,3.12 52.11,3.12 52.61,3.62 52.61,5.27 55.23,7.89 R30.2 | U24.49 63.5,25.36 67.63,29.49 | 68.23,16.94 U24.47 | LED1.- 4.07,26.02 J3.P$9 | C17.1 C2.1
  Top 0.8: 67.63,29.49 67.97,29.49 68.76,30.28 68.82,30.28 69.16,30.62 U24.1 69.16,29.67 68.16,28.67 | 69.16,16.01 68.23,16.94
  Top 1: 69.11,12.33 69.11,13.93 U24.38 69.16,16.01
  other vias: 36.71,38.54 3.55,3.53 15.14,43.71 51.92,29.73 12.74,37.95 15.71,38.09 3.55,43.26 73.3,43.26 46.68,43.79 67.03,20.09 67.13,23.74 67.08,27.79 46.33,5.74 64.58,16.74 60.53,17.34 26.73,4.64 20.46,6.05 41.45,37.1 33.09,11.93 55.71,38.18 52.56,37.62 22.28,4.64 17.83,28.54 12.31,28.8 36.47,32.77 44.63,33.09 9.03,36.79 11.13,17.49 11.11,20.07 38.49,28.01 65.13,41.49 49.78,40.24 8.98,40.04 34.73,39.94 19.08,28.54 58.68,40.09 16.6,42.93 31.33,43.69 61.43,26.29 66.43,38.09 36.93,5.79 65.13,33.34 67.73,38.14 35.87,33.92 63.73,26.29 21.63,21.39 30.54,27.74 28.71,28.13 19.14,37.83 22.24,16.73 18.99,10.68 20.49,3.73 15.1,29.14 8.66,25.63 50.61,13.72 29.49,9.93 8.73,10.07 33.83,11.34 40.99,16.46 16.09,21.08 35.04,4.53 11.39,24.13 11.14,27.48 29.3,16.83 26.84,9.98 50.94,34.58 29.49,11.13 30.58,10.67 49.64,33.33 8.71,24.13 23.83,39.57 26.3,35.91 8.71,17.46 8.8,11 9.64,10.95 8.71,37.8 9.78,37.84 9.08,35.64
  pour Bottom: 68.66,44.82 68.66,1.92 8.16,1.92 8.16,44.82
  pour Top (rank 2): -0.04,47.02 76.86,47.02 76.91,47.07 76.91,40.55 69.61,40.55 69.61,6.5 76.86,6.5 76.86,0.02 0.01,0.02 -0.04,-0.03
IN-
  Top 0.254: 67.06,6.07 66.89,6.07 65.03,6.07 U2.4 | R37.1 67.06,6.07 | R22.2 67.06,4.93 67.06,6.07
IO0_BOOT  (via drill 0.35)
  Top 0.254: U24.25 52.65,24.68 v52.74,24.78 | v15.01,41.17 14.36,41.17 K1.2 | v38.09,30.85 37.89,31.04 Q10.3
  Bottom 0.254: v52.74,24.78 43.07,24.78 38.09,29.76 v38.09,30.85 38.09,33.12 30.04,41.17 v15.01,41.17
IO2_TFT_RS  (via drill 0.35)
  Top 0.254: v46.93,19.64 49.5,17.06 U24.24
  Bottom 0.254: v46.93,19.64 46.74,19.83 26.27,19.83 J1.P$4
IO5_TF_CS
  Top 0.254: R67.2 37.29,16.25 SD1.2 37.29,13.13 37.71,12.72 57.24,12.72 57.74,13.22 57.74,13.97 U24.29
IO12_TFT_SDO/TP_OUT  (via drill 0.35)  (1 unrouted)
  Top 0.254: v55.16,18.13 55.11,18.18 55.11,27.61 52.65,30.07 U24.14 50.63,31.58 49.26,30.21 R2.1 | v18.13,18.75 18.13,17.07
  Bottom 0.254: v55.16,18.13 50.87,18.13 47.25,14.51 19.35,14.51 18.13,15.73 v18.13,18.75
IO13_TFT_SDI/TP_DIN  (via drill 0.35)
  Top 0.254: R29.1 41.43,21 41.63,21.2 v41.63,21.36 42.38,22.12 48.76,22.12 49.57,22.93 49.57,26.69 50.2,27.32 50.95,27.32 U24.16 | U3.14 19.38,19.34 v19.66,19.62
  Bottom 0.254: v41.63,21.36 41.63,21.28 J1.P$6 22.97,21.28 22.06,20.37 20.41,20.37 v19.66,19.62
IO14_TFT_CLK/TP_CLK  (via drill 0.35)
  Top 0.254: U24.13 53.92,29.93 55.84,28.01 v55.84,20.23 | R28.1 30.32,17.89 29.37,18.85 v29.14,18.85 | U3.16 20.65,17.62 21.5,18.47 v22.36,18.47
  Bottom 0.254: v55.84,20.23 55.78,20.29 50.19,20.29 48.64,18.74 29.24,18.74 v29.14,18.85 29.1,18.88 J1.P$3 22.77,18.88 v22.36,18.47
IO15_TFT_CS  (via drill 0.35)
  Top 0.254: v48.28,20.15 50.09,18.33 U24.23
  Bottom 0.254: v48.28,20.15 47.81,20.62 26.26,20.62 J1.P$5
IO16_RXD2  (via drill 0.35)
  Top 0.254: U24.27 55,14.17 55,15.09 53.47,16.61 v53.47,22.38 | v28.75,35.12 v28.76,35.12 28.76,37.04 J10.1
  Bottom 0.254: v53.47,22.38 53.31,22.55 40.06,22.55 28.75,33.86 v28.75,35.12
IO17_TXD2  (via drill 0.35)
  Top 0.254: U24.28 56.37,14.07 56.37,15.11 54.36,17.12 v54.36,23.57 | v30.72,35.14 30.74,35.14 J10.2
  Bottom 0.254: v30.72,35.14 30.72,33.61 40.76,23.57 v54.36,23.57
IO18_TF_SPI_CLK
  Top 0.254: U24.30 59.01,13.97 59.01,13.22 56.75,10.96 35.41,10.96 33.99,12.38 SD1.5
IO19_TF_SPI_MISO
  Top 0.254: R24.2 33.58,17.63 31.79,15.84 SD1.7 31.83,15.09 31.83,11.72 33.2,10.35 57.09,10.35 60.27,13.53 U24.31
IO21_SCL  (via drill 0.35)  (2 unrouted)
  Top 0.254: U24.33 62.81,19.06 v62.01,19.87 | R26.1 41.96,34.57 43.86,36.47
  Bottom 0.254: v62.01,19.87 62.01,20.46 55.41,27.05 44.72,27.05 41.96,29.82 41.96,32.74 v41.99,32.77
IO22_SDA  (via drill 0.35)  (3 unrouted)
  Top 0.254: U24.36 66.62,16.85 v63.41,20.07 | R27.1 43.44,33.85 45.51,35.92
  Bottom 0.254: v63.41,20.07 63.41,20.37 55.86,27.92 45.16,27.92 43.41,29.67 43.41,33.02
  other vias: 43.43,33.04
IO23_TF_SPI_MOSI  (via drill 0.35)
  Top 0.254: R23.2 36.19,16.47 SD1.3 36.19,12.38 36.81,11.77 v56.41,11.77 | U24.37 67.89,12.42 v67.48,12.02
  Bottom 0.254: v67.48,12.02 67.48,11.94 66.64,11.1 57.08,11.1 v56.41,11.77
IO25_PROT_A/D  (via drill 0.35)  (1 unrouted)
  Top 0.254: v57.69,30.12 57.73,30.16 U24.10 57.73,35.54 58.66,36.47 | R18.1 46.33,29.28 v46.44,29.16
  Bottom 0.254: v57.69,30.12 57.05,30.76 47.9,30.76 46.44,29.3 v46.44,29.16
IO26_SPEAK  (via drill 0.35)
  Top 0.254: U24.11 56.46,29.68 57.07,29.08 57.07,18.49 v59.6,15.96 | v63.18,12.46 63.28,12.36 63.28,11.5 R12.1
  Bottom 0.254: v63.18,12.46 59.68,15.96 v59.6,15.96
IO27_LCD_BLK_CTR  (via drill 0.35)  (1 unrouted)
  Top 0.254: U24.12 55.19,30.25 56.58,28.86 56.58,16.19 v56.92,15.85 | v14.95,23.39 13.9,23.39 12.48,21.96 Q6.1
  Bottom 0.254: v56.92,15.85 51.65,15.85 48.57,12.77 18.4,12.77 14.95,16.21 v14.95,23.39
IO32_PROT_A/D  (via drill 0.35)  (1 unrouted)
  Top 0.254: v60.11,29.57 60.27,29.73 U24.8 60.27,36.18 60.61,36.52 | v49.06,28.97 48.47,28.97 47.76,29.68 R1.1
  Bottom 0.254: v49.06,28.97 59.51,28.97 v60.11,29.57
IO33_TP_CS  (via drill 0.35)
  Top 0.254: U24.9 59,29.68 57.85,28.53 57.85,19.26 v57.79,19.2 | U3.15 20.01,18.05 v20.92,18.96
  Bottom 0.254: v57.79,19.2 50.42,19.2 46.76,15.54 21.35,15.54 20.92,15.96 20.92,17.37 v20.92,18.96
IO36_TP_IRQ  (via drill 0.35)
  Top 0.254: v58.61,18.02 58.52,18.1 58.52,26.08 60.78,28.33 63.48,28.33 65.35,30.2 U24.4 | R10.1 15.16,17.32 15.16,17.82 16.06,18.72 v16.76,18.72 17.38,18.09 17.47,18 U3.11
  Bottom 0.254: v58.61,18.02 57.57,16.98 51.58,16.98 48.25,13.65 18.86,13.65 16.75,15.76 16.76,15.77 v16.76,18.72
N$1
  Top 0.254: 2.11,22.53 LED1.+
  Top 1: R3.1 2.19,22.45 2.11,22.53
N$2
  Top 0.254: R7.2 12.48,18.82 14.26,20.6 Q6.3
N$3
  Top 0.254: R12.2 63.35,10 62.08,11.27 R19.1 C46.2
N$4
  Top 0.254: U3.7 16.84,23.45 15.78,24.51 R35.2
N$6
  Top 1: U26.5 8.22,21.97 R9.1
N$12  (via drill 0.35)  (2 unrouted)
  Top 0.254: R7.1 14.88,18.82 16.18,20.12 v17.56,20.12
  Bottom 0.254: J1.P$14 J1.P$11 | J1.P$11 | v17.56,20.12 17.66,20.12 22.81,25.27 J1.P$11
N$13  (1 unrouted)
  Top 0.8: U1.3 23.96,2.48
N$14
  Top 0.254: J3.B5 9.95,29.82 12.28,27.49 R33.1
N$16
  Top 0.254: J3.A5 8.31,32.84 9.33,32.84 9.54,33.05 9.54,34.4 10.96,35.82 R34.2
N$17
  Top 0.5: Q3.1 9.98,2.21 R6.2 R25.1
N$20
  Top 0.254: U1.5 17.78,4.88 20.42,7.53 R21.1 R20.2
N$26
  Top 0.254: C51.2 59.48,9.25 59.99,8.73 61.52,8.73 62.08,9.29 R19.2 62.08,9.66 64.04,7.7 68.72,7.7 70.06,6.37 70.06,3.92 69.61,3.47 C14.1
N$29
  Top 0.254: C14.2 68.55,4.76 R22.1
N$32
  Top 0.254: R75.1 29.13,30.41 Q9.1
N$38
  Top 0.3: R74.1 27.37,32.14 27.37,33.31 27.94,33.89 33.59,33.89 34.41,33.07 Q10.1
N$40  (via drill 0.35)
  Top 0.254: R72.2 64.65,9.36 v64.11,8.82 | U6.2 20.48,36.07 v20.48,34.97
  Bottom 0.254: v64.11,8.82 17.35,8.82 13.91,12.27 13.91,30.07 17.72,33.88 19.38,33.88 v20.48,34.97
N$42  (via drill 0.35)
  Top 0.254: R71.2 65.98,9.09 v65.61,8.72 | v19.06,34.92 U6.3
  Bottom 0.254: v65.61,8.72 65.61,8.07 64.86,7.32 17.46,7.32 13.06,11.72 13.06,30.75 17.22,34.92 v19.06,34.92
N$47
  Top 0.254: R16.2 39.9,17.68 39.9,17.14 38.39,15.63 SD1.1
N$48
  Top 0.254: SD1.8 30.69,15.93 32.22,17.46 R17.2
RTS  (via drill 0.35)
  Top 0.254: R74.2 26.19,31.79 v26.19,32.47 | v19.13,32.56 19.07,32.49 U6.14
  Top 0.3: R74.2 27.62,29.53 28.12,29.03 30.14,29.03 30.8,29.69 Q9.2
  Bottom 0.254: v26.19,32.47 26.11,32.56 v19.13,32.56
TFT_RESET  (via drill 0.35)
  Top 0.3: R8.1 C28.1 44.42,19.21 45.82,17.8 R5.1 45.82,16.74 v45.76,16.68
  Bottom 0.3: J1.P$2 26.2,17.99 44.45,17.99 v45.76,16.68
TP_X+  (via drill 0.35)
  Top 0.254: 21,24.49 C18.2 21.03,25.82 21.11,25.82 | 21,24.49 20.01,23.5 U3.2 | v22.01,25.82 21.11,25.82 | 21,24.49 21.11,24.6 21.11,25.82
  Bottom 0.254: J1.P$15 23.92,28.48 22.01,26.57 v22.01,25.82
TP_X-  (via drill 0.35)
  Top 0.254: C20.2 18.44,25.76 18.44,24.63 v18.58,24.49 18.74,24.33 U3.4
  Bottom 0.254: J1.P$17 23.21,30.08 20.51,27.37 20.51,24.53 20.01,24.03 19.04,24.03 v18.58,24.49
TP_Y+  (via drill 0.35)
  Top 0.254: C19.2 19.72,24.83 v19.68,24.79 19.66,24.77 19.42,24.53 19.38,24.49 U3.3
  Bottom 0.254: v19.68,24.79 19.68,27.69 22.87,30.87 J1.P$18
TP_Y-  (via drill 0.35)
  Top 0.254: C21.2 17.19,24.6 v17.28,24.51 18.11,23.68 U3.5
  Bottom 0.254: J1.P$16 23.27,29.28 21.01,27.02 21.01,24.15 20.28,23.41 18.38,23.41 v17.28,24.51 | v17.28,24.51
UART0_RXD0
  Top 0.254: R72.1 64.08,12 U24.34
UART0_TXD0
  Top 0.254: R71.1 65.35,12.06 U24.35
USB_D+
  Top 0.254: R32.2 11.2,31.59 12.83,33.22 14.81,33.22 16.53,34.93 U6.5
USB_D-
  Top 0.254: R11.2 11.56,32.87 12.56,33.87 14.66,33.87 15.25,34.46 U6.6
VBUS  (via drill 0.35)  (8 unrouted)
  Top 0.5: R25.2 8.46,8.53 9.05,9.12 v9.47,9.12
  Top 0.6: 8.14,29.17 7.19,29.17 | 7.99,33.97 7.23,33.97 | 8.45,29.17 9.36,29.17
  Top 0.65: 7.19,29.17 6.29,30.07 6.29,33.15 7.16,34.02 | 9.36,29.17 10.01,28.52
  Top 0.8: 16.57,13.3 17.21,13.3
  Top 1: 10.01,28.52 10.01,18.61 | 10.01,18.61 10.01,16 | 10.01,16 10.01,15.84 12.38,13.47 13,13.47 17.04,13.47 17.21,13.3 D3.1 | 10.01,16 9.67,16.34 v9.14,16.34 | 10.01,18.61 U26.4
  Bottom 0.5: v9.47,9.12 9.56,9.12 10.9,10.46 10.9,13.49 9.05,15.34 9.05,16.26 v9.14,16.34
VIN
  Top 0.5: U1.1 17.69,2.98 U1.4
  Top 0.65: D3.2 17.12,7.94 17.31,7.75 | C42.2 16.37,4.22 17.69,2.9 U1.1
  Top 1: 17.31,7.75 17.31,7.12 15.82,5.63 C42.2 15.43,3.84 C6.2 13.19,3.84 12.07,2.71 Q3.2 | D3.2 15.98,9.8 D2.C
VO1  (via drill 0.5)
  Top 0.254: v49.41,5.42 49.47,5.48 | U2.5 59.64,6.07 | 68.74,6.12 R37.2
  Top 0.5: J8.P$1 49.47,5.48 | 59.64,6.07 v58.37,6.07 | U2.5 60.66,7.04 67.82,7.04 68.74,6.12
  Bottom 0.5: v58.37,6.07 57.98,5.67 49.66,5.67 v49.41,5.42
VO2  (via drill 0.5)  (1 unrouted)
  Top 0.254: v61.53,2.79 60.98,2.23 U2.8 | 51.41,6.77 51.61,6.97
  Top 0.5: v51.41,4.22 51.41,6.77
  Bottom 0.5: v61.53,2.79 60.1,4.22 v51.41,4.22

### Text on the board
tPlace: 3V3 | IO16_RXD | IO17_TXD | 3V3 | GND | IO21_SCL | IO22_SDA | 3V3 | GND | IO25 | IO32 | GND | www.elecrow.com | + | V2.0 | IO26-SPK | VO1 | VO2 | -
tStop: ESP32 Display-2.4 Inch | SKU:DIS03024H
